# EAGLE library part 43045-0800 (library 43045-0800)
Micro-Fit 3.0 Right-Angle Header, 3.00mm Pitch, Dual Row, 8 Circuits, with Snap-in Plastic Peg PCB Lock Source: Datasheet
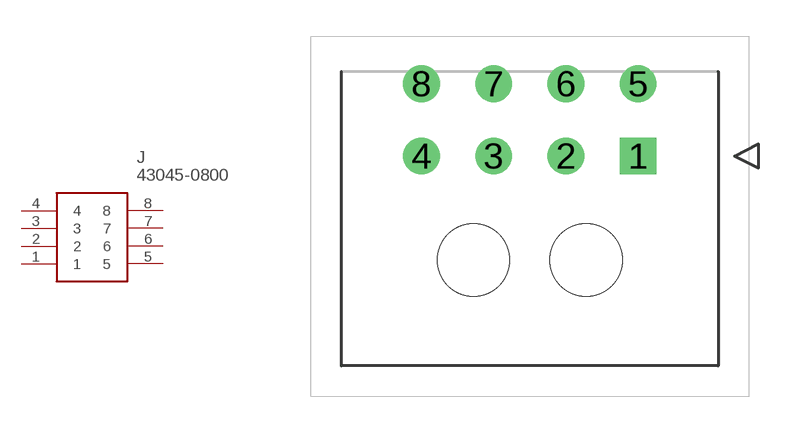
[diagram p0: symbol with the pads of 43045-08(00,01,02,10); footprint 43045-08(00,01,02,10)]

Designator prefix J

## 43045-0800 (Description: Micro-Fit 3.0 Right-Angle Header, 3.00mm Pitch, Dual Row, 8 Circuits, with Snap-in Plastic Peg PCB Lock; Height: 8.77mm; Manufacturer_Name: Molex; Manufacturer_Part_Number: 43045-0800; Mouser_Part_Number: 538-43045-0800; Mouser_Price-Stock: https://www.mouser.co.uk/ProductDetail/Molex/43045-0800?qs=MGlPTwjtJ4Z70Z3DbkGxKw%3D%3D)  [43045-08(00,01,02,10)]
1  1
2  2
3  3
4  4
5  5
6  6
7  7
8  8

## Footprint 43045-08(00,01,02,10) (pad centres in mm)
43045-08(00,01,02,10)
drill 1.02 pad 1.52 square: 1 0,0
drill 1.02 pad 1.52: 2 -3,0; 3 -6,0; 4 -9,0; 5 0,3; 6 -3,3; 7 -6,3; 8 -9,3
hole 3 at -2.16,-4.32
hole 3 at -6.84,-4.32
